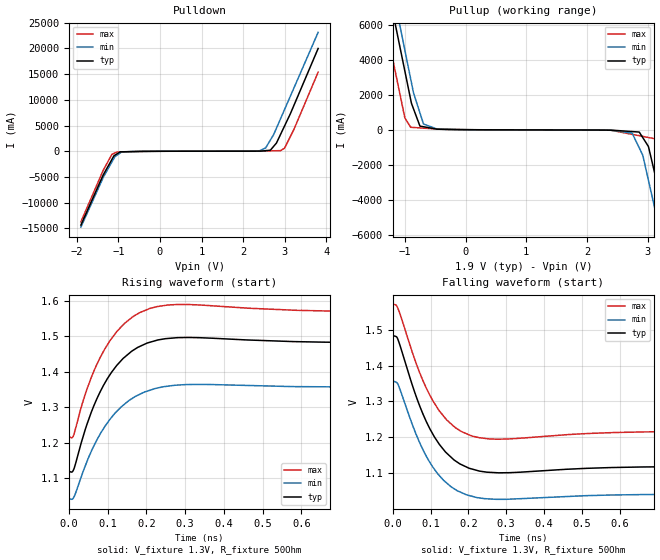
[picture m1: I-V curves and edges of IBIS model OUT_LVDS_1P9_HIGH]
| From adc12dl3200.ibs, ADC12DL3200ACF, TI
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|   OUT_LVDS_1P9_HIGH
[Model]   OUT_LVDS_1P9_HIGH
Model_type   Output
Polarity   Non-Inverting
Vmeas = 1.3
Vref = 1.3
Cref = 2pF
Rref = 50
|   typ   min   max
C_comp   1.674E-12   1.548E-12   1.744E-12
[Voltage Range]   1.9   1.8   2
[Temperature Range]   90   150   -55
[Pullup Reference]   1.9   1.8   2
[Pulldown Reference]   -0   0   -0
[Power Clamp Reference]   1.9   1.8   2
[GND Clamp Reference]   0   0   0
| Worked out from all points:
|   slope of the pulldown table from 0 to 0.285 V, typ, clamps not added: 42.5 ohm
|   slope of the pullup table from 0 to 0.285 V, typ, clamps not added: 46.4 ohm
|   falling waveform, V_fixture 1.3V, R_fixture 50Ohm: 20-80 % time 83.5ps typ, 82.4ps min, 82.2ps max; typ from 1.48 V to 1.12 V
|   rising waveform, V_fixture 1.3V, R_fixture 50Ohm: 20-80 % time 87.8ps typ, 96ps min, 85.3ps max; typ from 1.12 V to 1.48 V
[Pulldown]
|   Voltage   I(typ)   I(min)   I(max)
-1.9V     -14.37A    -14.78A    -13.74A
-1.362V   -4.603A    -5.097A    -3.689A
-1.157V   -1.623A    -2.116A    -633.4mA
-1.079V   -747.5mA   -1.027A    -323.3mA
-916.3mV  -114.2mA   -128.1mA   -128mA
2.31V     17.06mA    24.21mA    13.83mA
2.54V     112.8mA    652.1mA    43.13mA
2.653V    200.4mA    2.177A     66.36mA
2.796V    1.57A      4.452A     95.91mA
2.996V    4.965A     8.173A     626mA
3.222V    9.002A     12.38A     4.328A
3.8V      20A        23.14A     15.39A
[Pullup]
|   Voltage   I(typ)   I(min)   I(max)
-1.9V     20A        21.21A     17.34A
-1.222V   7.102A     8.351A     4.385A
-1.004V   3.393A     4.596A     718mA
-905.8mV  1.735A     2.916A     141.2mA
-694.3mV  171.3mA    330.6mA    91.55mA
-464mV    31.89mA    32.08mA    37.53mA
2.744V    -104.2mA   -192mA     -263.9mA
3.01V     -941mA     -2.844A    -441.6mA
3.145V    -2.911A    -4.921A    -532.2mA
3.223V    -4.062A    -6.118A    -1.634A
3.346V    -6.097A    -8.364A    -3.406A
3.8V      -14.37A    -16.65A    -11.82A
[Ramp]
R_load = 50
|   typ   min   max
dV/dt_r   0.217788/8.79142e-11   0.188664/9.6117e-11   0.211851/8.53163e-11
dV/dt_f   0.21779/8.35074e-11   0.188664/8.24312e-11   0.211844/8.22177e-11
[Falling Waveform]
V_fixture = 1.3V
V_fixture_min = 1.2V
V_fixture_max = 1.4V
R_fixture = 50Ohm
C_fixture = 0F
|   Time   V(typ)   V(min)   V(max)
0s        1.482V     1.356V     1.57V
12.75ps   1.475V     1.35V      1.561V
71.72ps   1.286V     1.184V     1.379V
98.54ps   1.223V     1.13V      1.317V
123.2ps   1.181V     1.094V     1.274V
155.1ps   1.144V     1.062V     1.237V
182.1ps   1.124V     1.046V     1.216V
249ps     1.103V     1.029V     1.196V
762.6ps   1.119V     1.042V     1.216V
5ns       1.119V     1.042V     1.217V
[Rising Waveform]
V_fixture = 1.3V
V_fixture_min = 1.2V
V_fixture_max = 1.4V
R_fixture = 50Ohm
C_fixture = 0F
|   Time   V(typ)   V(min)   V(max)
0s        1.119V     1.042V     1.217V
11.83ps   1.124V     1.045V     1.22V
41.7ps    1.236V     1.133V     1.336V
70.6ps    1.32V      1.205V     1.418V
98.54ps   1.379V     1.255V     1.475V
123.2ps   1.418V     1.288V     1.513V
182.1ps   1.471V     1.336V     1.567V
280.4ps   1.496V     1.362V     1.59V
880.2ps   1.482V     1.356V     1.57V
5ns       1.482V     1.356V     1.57V
